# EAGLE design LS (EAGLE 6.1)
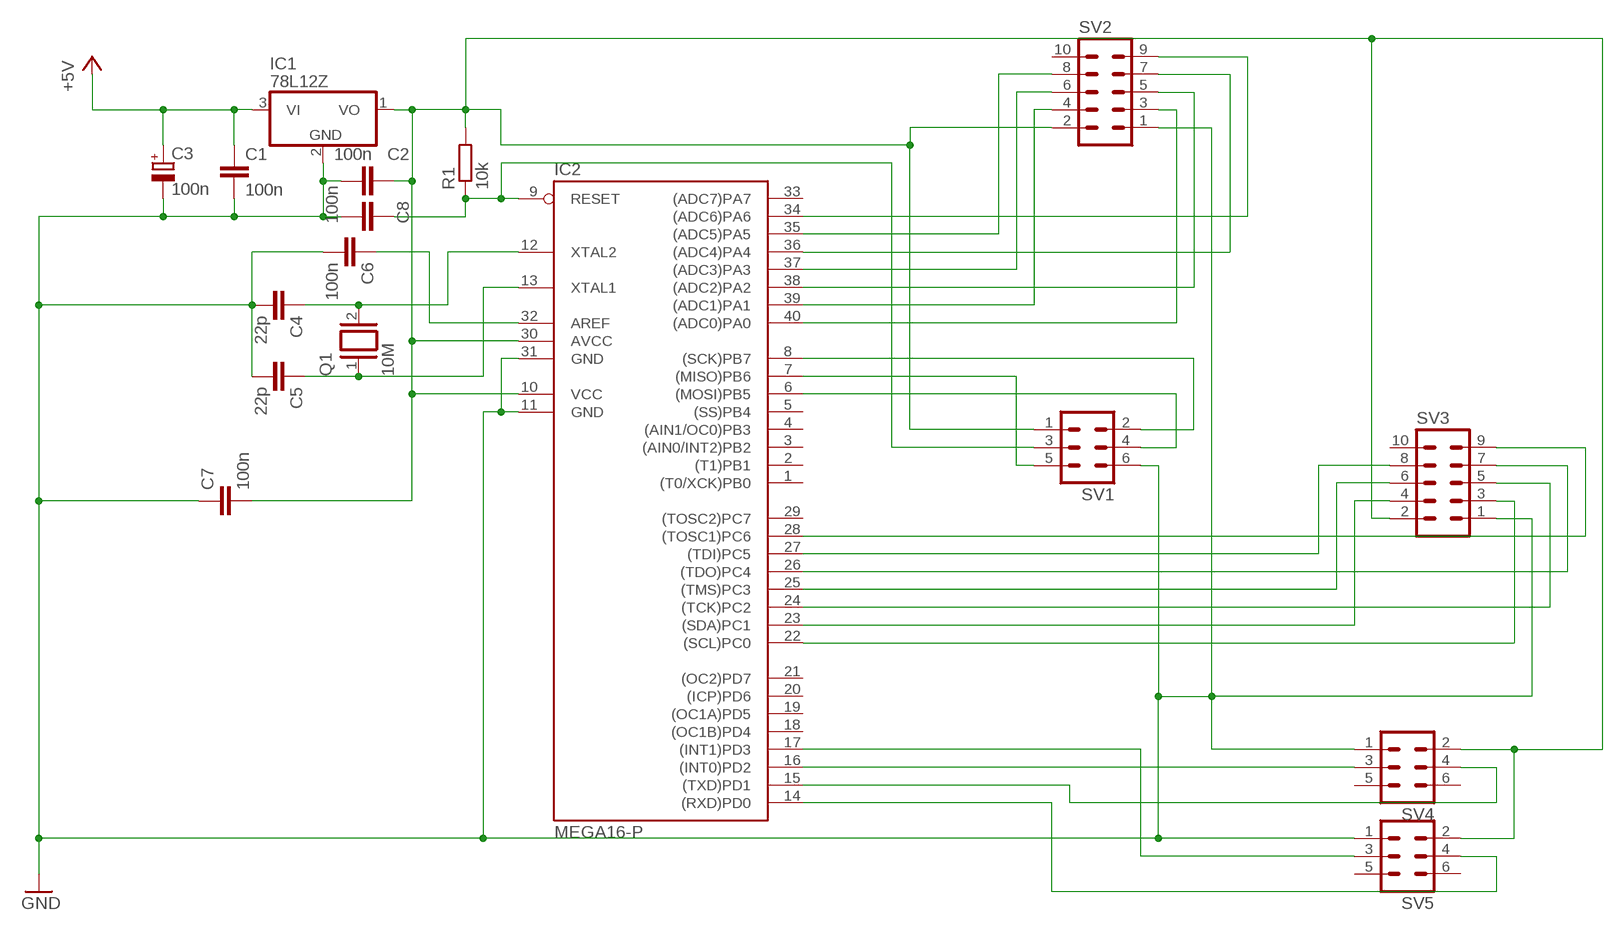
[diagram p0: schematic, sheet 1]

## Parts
C1  100n  C-EU075-032X103  [C075-032X103]
C2  100n  C-EU075-032X103  [C075-032X103]
C3  100n  CPOL-EUE2.5-7  [E2,5-7]
C4  22p  C-EU075-032X103  [C075-032X103]
C5  22p  C-EU075-032X103  [C075-032X103]
C6  100n  C-EU075-052X106  [C075-052X106]
C7  100n  C-EU075-032X103  [C075-032X103]
C8  100n  C-EU075-032X103  [C075-032X103]
IC1  78L12Z  [TO92]
IC2  MEGA16-P  [DIL40]
Q1  10M  XTAL/S  [QS]
R1  10k  R-EU_0207/10  [0207/10]
SV1  ML6  [ML6]
SV2  ML10  [ML10]
SV3  ML10  [ML10]
SV4  ML6  [ML6]
SV5  ML6  [ML6]

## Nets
+5V: C1.1 C3.+ IC1.3(VI)
GND: C1.2 C2.2 C3.- C4.2 C5.2 C6.2 C7.1 C8.1 IC1.2(GND) IC2.11(GND) IC2.31(GND) SV1.6 SV2.1 SV3.1 SV4.1 SV5.1
N$1: C6.1 IC2.32(AREF)
N$2: IC2.22((SCL)PC0) SV3.3
N$3: IC2.23((SDA)PC1) SV3.4
N$4: C8.2 IC2.9(RESET) R1.1 SV1.3
N$5: IC2.24((TCK)PC2) SV3.5
N$6: IC2.7((MISO)PB6) SV1.5
N$7: IC2.6((MOSI)PB5) SV1.4
N$8: C4.1 IC2.12(XTAL2) Q1.2
N$9: C5.1 IC2.13(XTAL1) Q1.1
N$10: IC2.8((SCK)PB7) SV1.2
N$11: IC2.40((ADC0)PA0) SV2.3
N$12: C2.1 C7.2 IC1.1(VO) IC2.10(VCC) IC2.30(AVCC) R1.2 SV1.1 SV2.2 SV3.2 SV4.2 SV5.2
N$13: IC2.39((ADC1)PA1) SV2.4
N$14: IC2.25((TMS)PC3) SV3.6
N$15: IC2.38((ADC2)PA2) SV2.5
N$16: IC2.37((ADC3)PA3) SV2.6
N$17: IC2.36((ADC4)PA4) SV2.7
N$18: IC2.35((ADC5)PA5) SV2.8
N$19: IC2.26((TDO)PC4) SV3.7
N$20: IC2.27((TDI)PC5) SV3.8
N$21: IC2.28((TOSC1)PC6) SV3.9
N$22: IC2.34((ADC6)PA6) SV2.9
N$23: IC2.15((TXD)PD1) SV4.4
N$24: IC2.14((RXD)PD0) SV5.4
N$25: IC2.16((INT0)PD2) SV4.3
N$26: IC2.17((INT1)PD3) SV5.3
Unconnected: IC2.1((T0/XCK)PB0) IC2.2((T1)PB1) IC2.3((AIN0/INT2)PB2) IC2.4((AIN1/OC0)PB3) IC2.5((SS)PB4) IC2.18((OC1B)PD4) IC2.19((OC1A)PD5) IC2.20((ICP)PD6) IC2.21((OC2)PD7) IC2.29((TOSC2)PC7) IC2.33((ADC7)PA7) SV2.10 SV3.10 SV4.5 SV4.6 SV5.5 SV5.6

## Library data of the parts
C1 C2 C4-C8 = rcl:C-EU: CAPACITOR, European symbol
C3 = rcl:CPOL-EU: POLARIZED CAPACITOR, European symbol
IC1 = linear:78*: Positive VOLTAGE REGULATOR Source: http://cache.national.com/ds/LM/LM78L05.pdf http://www.fairchildsemi.com/ds/LM/LM7805.pdf
IC2 = atmel:MEGA16-P: MICROCONTROLLER 16 Kbytes FLASH 1 kbytes SRAM 512 bytes EEPROM USART 8-channel 10 bit ADC Source: avr.lbr; MPN: ATMEGA16-16PU; OC_FARNELL: 9171142; OC_NEWARK: 01M6885
Q1 = special:XTAL/S: CRYSTAL
R1 = rcl:R-EU_: RESISTOR, European symbol
SV1 SV4 SV5 = con-harting-ml:ML6: HARTING; OC_FARNELL: unknown; OC_NEWARK: unknown
SV2 SV3 = con-harting-ml:ML10: HARTING; OC_FARNELL: unknown; OC_NEWARK: unknown

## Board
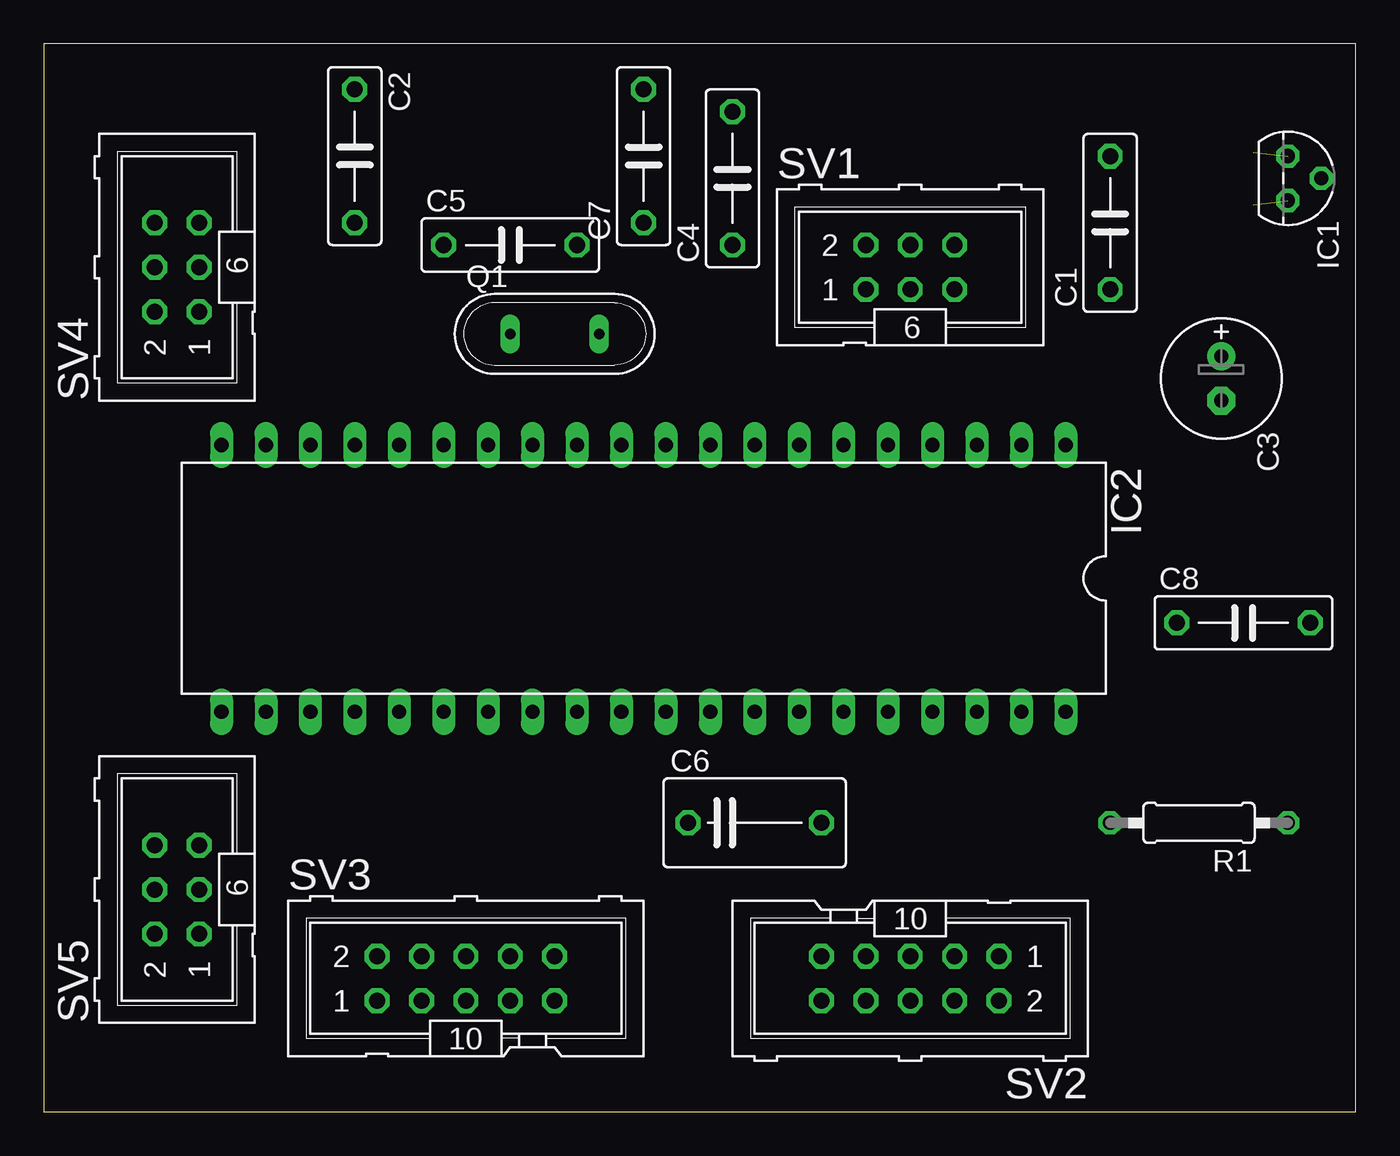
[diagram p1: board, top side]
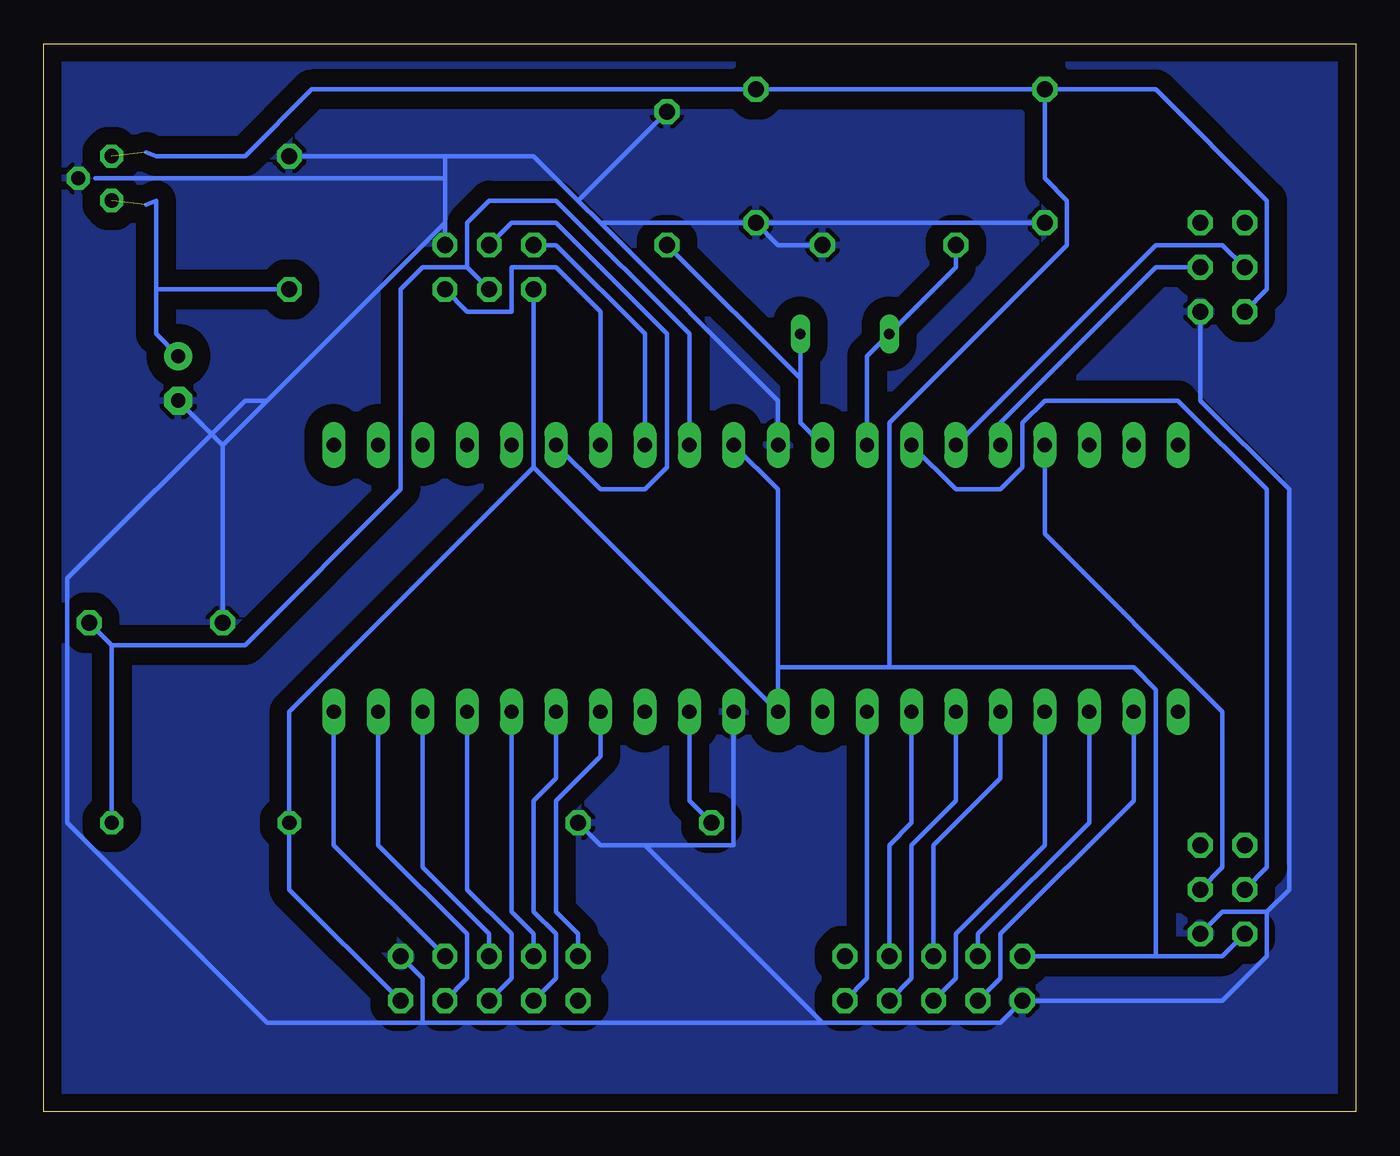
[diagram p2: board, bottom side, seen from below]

Size 75 x 61.03 mm. Coordinates in mm from the lower left corner, seen from the top.
Outline: 0,0 75,0 75,61.03 0,61.03 0,0
Copper layers (1*16): Top 0.035mm / dielectric 1.5mm / Bottom 0.035mm
Design rules: minimum track width 10mil, minimum drill 24mil, track to track 8mil, track to pad 8mil, pad to pad 8mil, via to via 8mil, smd to smd 8mil, copper to edge 40mil, drill to drill 8mil, minimum pad ring 10mil, minimum via ring 8mil, stop-mask expansion 4mil, vias tented up to drill 0mil, thermal gap 10mil

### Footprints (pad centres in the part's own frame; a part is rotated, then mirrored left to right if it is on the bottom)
C075-032X103 = drill 0.914 octagon: 1 -3.81,0; 2 3.81,0
E2,5-7 = drill 0.813 pad 1.6: + -1.27,0 | drill 0.813 pad 1.6 octagon: - 1.27,0
C075-052X106 = drill 0.914 octagon: 1 -3.81,0; 2 3.81,0
TO92 = drill 0.813 octagon: 1 -1.27,0; 2 0,1.905; 3 1.27,0
DIL40 = drill 0.813 long: 1 -24.13,-7.62; 2 -21.59,-7.62; 3 -19.05,-7.62; 4 -16.51,-7.62; 5 -13.97,-7.62; 6 -11.43,-7.62; 7 -8.89,-7.62; 8 -6.35,-7.62; 9 -3.81,-7.62; 10 -1.27,-7.62; 11 1.27,-7.62; 12 3.81,-7.62; 13 6.35,-7.62; 14 8.89,-7.62; 15 11.43,-7.62; 16 13.97,-7.62; 17 16.51,-7.62; 18 19.05,-7.62; 19 21.59,-7.62; 20 24.13,-7.62; 21 24.13,7.62; 22 21.59,7.62; 23 19.05,7.62; 24 16.51,7.62; 25 13.97,7.62; 26 11.43,7.62; 27 8.89,7.62; 28 6.35,7.62; 29 3.81,7.62; 30 1.27,7.62; 31 -1.27,7.62; 32 -3.81,7.62; 33 -6.35,7.62; 34 -8.89,7.62; 35 -11.43,7.62; 36 -13.97,7.62; 37 -16.51,7.62; 38 -19.05,7.62; 39 -21.59,7.62; 40 -24.13,7.62
QS = drill 0.61 long: 1 -2.54,0; 2 2.54,0
0207/10 = drill 0.813 octagon: 1 -5.08,0; 2 5.08,0
ML6 = drill 0.914 octagon: 1 -2.54,-1.27; 2 -2.54,1.27; 3 0,-1.27; 4 0,1.27; 5 2.54,-1.27; 6 2.54,1.27
ML10 = drill 0.914 octagon: 1 -5.08,-1.27; 2 -5.08,1.27; 3 -2.54,-1.27; 4 -2.54,1.27; 5 0,-1.27; 6 0,1.27; 7 2.54,-1.27; 8 2.54,1.27; 9 5.08,-1.27; 10 5.08,1.27

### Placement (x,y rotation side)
C1  60.96,50.8 90 top
C2  17.78,54.61 270 top
C3  67.31,41.91 270 top
C4  39.37,53.34 90 top
C5  26.67,49.53 0 top
C6  40.64,16.51 0 top
C7  34.29,54.61 90 top
C8  68.58,27.94 0 top
IC1  71.12,53.34 270 top
IC2  34.29,30.48 180 top
Q1  29.21,44.45 0 top
R1  66.04,16.51 180 top
SV1  49.53,48.26 0 top
SV2  49.53,7.62 180 top
SV3  24.13,7.62 0 top
SV4  7.62,48.26 90 top
SV5  7.62,12.7 90 top

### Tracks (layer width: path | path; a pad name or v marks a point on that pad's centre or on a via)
+5V  (1 unrouted)
  Bottom 0.254: 68.58,46.99 68.58,44.45 C3.+ | 68.58,46.99 68.58,52.07 69.14,51.84 | 68.58,46.99 C1.1
GND
  Bottom 0.254: C5.2 33.02,49.53 C7.1 | C7.1 C2.2 | 64.77,38.1 C8.1 | C3.- 64.77,38.1 | IC2.11 33.02,40.64 43.18,50.8 | 44.45,52.07 46.99,54.61 52.07,54.61 | 44.45,52.07 43.18,50.8 | C1.2 52.07,54.61 | 52.07,54.61 52.07,53.34 | 52.07,53.34 52.07,50.8 | 52.07,50.8 SV1.6 | 44.45,52.07 C4.2 | 52.07,53.34 72.06,53.34 | 52.07,50.8 62.23,40.64 | 62.23,40.64 64.77,38.1 | 43.18,50.8 C7.1 | IC2.31 35.56,15.24 40.64,15.24 | 40.64,15.24 43.18,15.24 C6.2 | 30.48,5.08 20.32,5.08 SV3.1 7.62,6.35 5.08,8.89 5.08,11.43 | 40.64,15.24 30.48,5.08 | SV2.1 53.34,7.62 53.34,5.08 | 30.48,5.08 53.34,5.08 | SV5.1 7.62,11.43 5.08,11.43 | SV4.1 8.89,40.64 3.81,35.56 3.81,12.7 5.08,11.43 | 62.23,40.64 63.5,40.64 73.66,30.48 73.66,16.51 62.23,5.08 53.34,5.08
  pour Bottom (isolate 1.016): -3.81,-3.81 -3.81,64.77 80.01,64.77 80.01,30.48 80.01,-6.35 -3.81,-6.35
N$1
  Bottom 0.254: IC2.32 38.1,17.78 C6.1
N$2
  Bottom 0.254: IC2.22 12.7,17.78 20.32,10.16 20.32,7.62 SV3.3
N$3
  Bottom 0.254: IC2.23 15.24,16.51 21.59,10.16 SV3.4
N$4
  Bottom 0.254: 71.12,26.67 R1.1 | C8.2 71.12,26.67 | IC2.9 38.1,44.45 45.72,52.07 49.53,52.07 50.8,50.8 50.8,48.26 | SV1.3 50.8,48.26 | 71.12,26.67 63.5,26.67 54.61,35.56 54.61,46.99 53.34,48.26 50.8,48.26
N$5
  Bottom 0.254: IC2.24 17.78,15.24 22.86,10.16 22.86,7.62 SV3.5
N$6
  Bottom 0.254: IC2.7 43.18,45.72 45.72,48.26 48.26,48.26 48.26,45.72 50.8,45.72 SV1.5
N$7
  Bottom 0.254: IC2.6 43.18,35.56 40.64,35.56 39.37,36.83 39.37,44.45 45.72,50.8 48.26,50.8 SV1.4
N$8
  Bottom 0.254: 31.75,41.91 31.75,39.37 IC2.12 | 31.75,41.91 Q1.2 | 31.75,41.91 C4.1
N$9
  Bottom 0.254: C5.1 22.86,48.26 Q1.1 27.94,43.18 IC2.13
N$10
  Bottom 0.254: IC2.8 40.64,44.45 45.72,49.53 SV1.2
N$11
  Bottom 0.254: IC2.40 58.42,15.24 SV2.3
N$12  (1 unrouted)
  Bottom 0.254: SV4.2 5.08,46.99 5.08,52.07 11.43,58.42 C2.1 | 69.14,54.84 68.58,54.61 63.5,54.61 59.69,58.42 C7.2 C2.1 | SV2.2 60.96,12.7 R1.2 60.96,22.86 46.99,36.83 | SV5.2 7.62,8.89 11.43,8.89 | SV3.2 11.43,8.89 | 33.02,25.4 33.02,35.56 IC2.10 | 33.02,25.4 IC2.30 46.99,36.83 | 46.99,36.83 SV1.1 | 11.43,8.89 11.43,24.13 12.7,25.4 26.67,25.4 | 33.02,25.4 26.67,25.4 | C2.1 17.78,53.34 16.51,52.07 16.51,49.53 26.67,39.37 26.67,25.4
N$13
  Bottom 0.254: IC2.39 55.88,15.24 50.8,10.16 50.8,7.62 SV2.4
N$14
  Bottom 0.254: IC2.25 20.32,19.05 24.13,15.24 SV3.6
N$15
  Bottom 0.254: IC2.38 53.34,13.97 49.53,10.16 SV2.5
N$16
  Bottom 0.254: IC2.37 50.8,12.7 48.26,10.16 48.26,7.62 SV2.6
N$17
  Bottom 0.254: IC2.36 48.26,11.43 46.99,10.16 SV2.7
N$18
  Bottom 0.254: IC2.35 45.72,19.05 46.99,17.78 46.99,11.43 45.72,10.16 45.72,7.62 SV2.8
N$19
  Bottom 0.254: IC2.26 22.86,17.78 25.4,15.24 25.4,7.62 SV3.7
N$20
  Bottom 0.254: IC2.27 25.4,16.51 26.67,15.24 SV3.8
N$21
  Bottom 0.254: IC2.28 27.94,7.62 SV3.9
N$22
  Bottom 0.254: IC2.34 43.18,20.32 45.72,17.78 45.72,11.43 44.45,10.16 SV2.9
N$23
  Bottom 0.254: IC2.15 11.43,49.53 7.62,49.53 SV4.4
N$24
  Bottom 0.254: IC2.14 22.86,35.56 20.32,35.56 19.05,36.83 19.05,39.37 17.78,40.64 10.16,40.64 5.08,35.56 5.08,13.97 SV5.4
N$25
  Bottom 0.254: IC2.16 20.32,39.37 11.43,48.26 SV4.3
N$26
  Bottom 0.254: IC2.17 17.78,33.02 7.62,22.86 7.62,13.97 SV5.3

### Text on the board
tRestrict: LS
